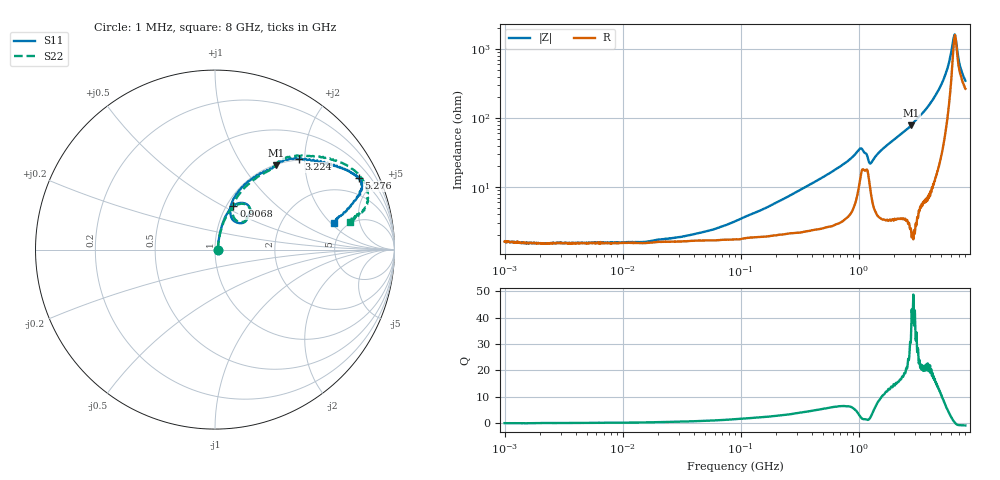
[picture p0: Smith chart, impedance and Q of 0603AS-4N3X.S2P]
!s-Parameter Generated by FASTRON Sdn. Bhd.
!FASTRON P/N : 0603AS-4N3X
!Keysight Technologies: E5071C_MY46733604_B.14.02
!Date: Tue Oct 24 10:26:25 2023
!Version  :Rev01  Tue Oct 24 10:26:25 2023
!Data & Calibration Information:
!Freq  S11:SOLT2(ON)  S21:SOLT2(ON)  S12:SOLT2(ON)  S22:SOLT2(ON)
!PortZ  Port1:50+j0  Port2:50+j0
!When reading reference impedance value at option line is always used.
! Remarks : This data is being provided solely for informational purposes.
# Hz S dB R 50
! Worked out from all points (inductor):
!   1601 points, 1 MHz to 8 GHz, reference 50 ohm
!   read as one part in series: L = 4.4 nH near 220.2 MHz
!   highest Q = 34.9 at 2.78 GHz (marker M1), where L = 4.51 nH
!   self-resonance near 6.568 GHz
!   S11 on the Smith chart (normalised r, x): 1 MHz: 1.03, -0.00; 906.8 MHz: 1.08, +0.56; 3.224 GHz: 0.98, +1.87; 5.276 GHz: 1.01, +4.00; 8 GHz: 3.95, +2.19
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1000000  -35.71 -0.9  -0.13 -0.1  -0.14 0.0  -35.75 1.0
2286470  -36.36 4.9  -0.14 -0.0  -0.14 -0.1  -37.24 4.9
4479405  -36.42 5.9  -0.14 -0.1  -0.14 -0.1  -36.82 6.5
1.518223e7  -37.70 8.8  -0.13 -0.3  -0.15 -0.3  -35.48 14.0
2.00676e7  -35.65 20.8  -0.14 -0.4  -0.15 -0.3  -35.43 24.2
5.02586e7  -33.25 43.7  -0.15 -0.9  -0.15 -0.9  -33.09 39.4
8.994653e7  -30.19 56.4  -0.15 -1.6  -0.16 -1.5  -30.36 54.7
4.006501e8  -19.15 73.5  -0.27 -6.1  -0.28 -6.1  -19.14 72.8
9.068124e8  -11.58 67.2  -0.80 -14.7  -0.80 -14.7  -11.58 65.8
1.041574e9  -10.28 51.9  -1.65 -15.8  -1.65 -15.8  -10.39 50.5
1.256741e9  -14.21 60.5  -0.98 -10.1  -0.98 -10.1  -13.84 57.2
1.7949e9  -8.42 66.6  -1.11 -22.0  -1.12 -22.1  -8.42 64.7
2.780342e9  -4.74 54.3  -2.89 -37.8  -2.91 -37.9  -4.84 54.6
3.223742e9  -3.25 47.2  -4.03 -41.3  -4.04 -41.3  -3.25 49.3
4.115571e9  -1.79 35.5  -6.89 -51.5  -6.88 -51.6  -1.75 38.5
5.276366e9  -0.98 26.5  -12.85 -56.8  -12.84 -56.9  -0.87 27.4
5.64026e9  -0.94 25.1  -15.68 -55.0  -15.67 -55.1  -0.80 24.8
6.265031e9  -1.08 22.5  -23.22 -31.5  -23.21 -31.7  -0.88 20.1
6.457806e9  -1.24 21.7  -25.46 -4.1  -25.45 -4.3  -0.96 18.6
6.689135e9  -1.43 20.2  -23.53 35.3  -23.52 35.0  -1.13 16.3
7.306013e9  -2.28 16.9  -16.53 50.2  -16.52 49.8  -1.89 14.0
8e9  -3.37 12.8  -13.53 49.3  -13.53 48.8  -2.30 11.6
